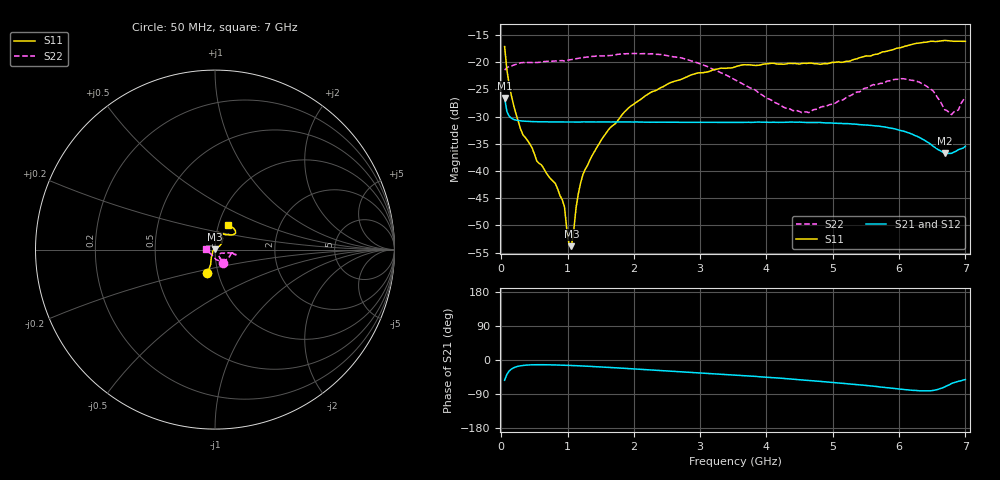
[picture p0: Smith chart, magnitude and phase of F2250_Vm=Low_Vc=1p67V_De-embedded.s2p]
! Integrated Device Technology
! Corporate Headquarters
! 6024 Silver Creek Valley Road
! San Jose, CA 95138  USA
! Phone:  1-408-284-8200
! Toll Free:  1-800-223-1366
! Webpage:  http://www.idt.com/
! Timing and RF Division
! 515 Groton Road, Suite 102
! Westford, MA 01886-6024
! Device:  F2250
! Description: Voltage Variable RF Attenuator
! Frequency:  50.0 -  6000.00 MHz
! Package:  3x3 mm Thin QFN Plastic Package: 16 pin
! Ports:  2 RF, 3 DC
!  Pin  1  = GND
!  Pin  2  = NC
!  Pin  3  = RF1  = Port 1
!  Pin  4  = NC
!  Pin  5  = GND
!  Pin  6  = GND
!  Pin  7  = GND
!  Pin  8  = GND
!  Pin  9  = NC
!  Pin 10  = RF2  = Port 2
!  Pin 11  = NC
!  Pin 12  = GND
!  Pin 13  = GND
!  Pin 14  = VCNTRL
!  Pin 15  = VDD
!  Pin 16  = VMODE
! Vcntrl:  1.670 Volts
! Vmode:  +0.000 Volts
! Vdd:  +3.30  Volts
! Current:  1.188 mA
! Data:  The device was measured on a the F2250 evaluation board which has
!  individual transmission lines to the RF pins.  Data was collected
!  using a calibrated network analyzer.  The evaluation board was
!  de-embedded using a TRL calibration technique.
!  The reference plane is the edge of the package pin.
! Misc:  SN 10
!  Action Tracker AT0258
! Date Measured:  2014-11-26
! Date:  2015-10-15  MJV
! Note:
!  Integrated Device Technology supplies this data as a sample of measured
!  data at the package pin for this product.  Your particular data for this
!  product may vary.
!  Data was taken at 25 degrees C.
!  Integrated Device Technology reserves the right to change this data at anytime.
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# GHz S dB R 50
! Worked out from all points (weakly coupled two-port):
!   201 points, 50 MHz to 7 GHz, reference 50 ohm
!   highest |S21| = -26.60 dB at 50 MHz (marker M1); lowest = -36.8 dB at 6.687 GHz (marker M2)
!   lowest |S11| = -53.8 dB at 1.058 GHz (marker M3), VSWR 1.00, Z = 50 + j0.198 ohm
!   |S11| at or under -10 dB: start of sweep to end of sweep
!   |S22| runs from -29.7 to -18.4 dB; largest |S21 - S12| = 0.00015
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0.05  -17.15 -107.8  -26.60 -53.4  -26.63 -53.4  -21.45 -60.0
0.1195  -24.20 -110.5  -29.94 -28.9  -29.93 -28.9  -20.83 -18.2
0.29325  -32.37 -125.1  -30.80 -15.2  -30.78 -15.2  -20.12 -9.7
0.5365  -38.19 -152.2  -30.95 -12.5  -30.96 -12.5  -20.06 -8.1
0.84925  -43.27 171.7  -31.01 -13.3  -31.02 -13.2  -19.78 -11.2
0.9535  -46.62 172.1  -31.00 -13.8  -31.01 -13.8  -19.80 -12.1
1.023  -53.62 135.4  -31.01 -14.2  -31.01 -14.2  -19.59 -12.0
1.05775  -53.82 103.0  -31.01 -14.5  -30.99 -14.5  -19.53 -12.1
1.162  -44.17 45.8  -31.01 -15.2  -30.98 -15.2  -19.29 -13.4
1.2315  -40.65 37.7  -30.98 -15.8  -30.99 -15.8  -19.17 -14.1
1.6485  -31.98 39.5  -31.00 -19.8  -31.01 -19.8  -18.80 -14.1
1.9265  -28.34 39.8  -30.99 -22.7  -30.99 -22.7  -18.45 -14.2
2.37825  -24.87 46.2  -31.03 -27.4  -31.03 -27.4  -18.58 -13.1
3.525  -20.88 71.9  -31.07 -40.0  -31.10 -39.9  -23.27 -16.8
4.2895  -20.35 76.8  -31.05 -48.9  -31.05 -49.0  -28.44 -33.7
4.7065  -20.26 72.1  -31.08 -54.9  -31.11 -54.9  -28.75 -49.5
5.85325  -17.87 40.1  -32.09 -73.7  -32.09 -73.8  -23.43 -62.2
6.305  -16.50 40.3  -33.82 -81.3  -33.83 -81.3  -23.68 -71.2
6.5135  -16.18 44.2  -35.46 -80.3  -35.46 -80.3  -25.29 -85.5
6.68725  -16.02 48.5  -36.79 -71.0  -36.76 -70.9  -28.74 -111.9
6.7915  -16.13 52.0  -36.76 -61.9  -36.74 -62.0  -29.65 -137.5
7  -16.18 63.0  -35.46 -51.4  -35.46 -51.4  -26.43 178.7
